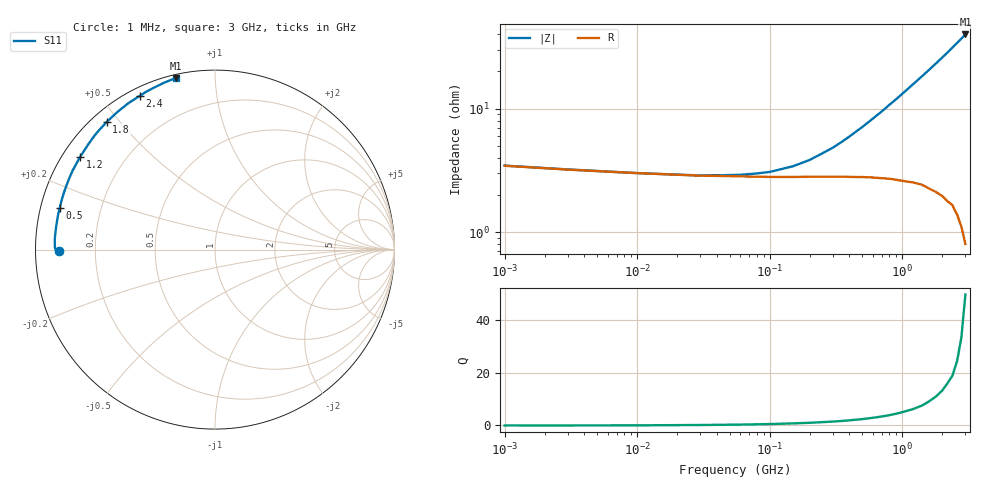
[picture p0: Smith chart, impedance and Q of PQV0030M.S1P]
! SIEMENS Small Signal Semiconductors
! BAR64-04
! Si PIN Diode in SOT23 (2 diodes in series, pin 3 open)
! IF = 30 mA
! S-Parameters:  July  1992
# GHz  S  MA  R  50
!  f  S11
! GHz  MAG  ANG
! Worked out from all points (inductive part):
!   33 points, 1 MHz to 3 GHz, reference 50 ohm
!   read as one part to ground: L = 2.05 nH near 700 MHz
!   highest Q = 49.8 at 3 GHz (marker M1), where L = 2.11 nH
!   S11 on the Smith chart (normalised r, x): 1 MHz: 0.07, -0.01; 500 MHz: 0.06, +0.13; 1.2 GHz: 0.05, +0.31; 1.8 GHz: 0.04, +0.46; 2.4 GHz: 0.03, +0.62; 3 GHz: 0.02, +0.80
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0.001  0.8712 -179.4
0.003  0.8796 -179.4
0.01  0.8868 -179.8
0.03  0.8918 179.4
0.08  0.8937 177.7
0.15  0.8944 175.5
0.2  0.8941 174.0
0.25  0.8941 172.4
0.3  0.8942 171.0
0.4  0.8952 168.0
0.45  0.8957 166.5
0.5  0.896 165.1
0.6  0.8976 162.2
0.7  0.8996 159.4
0.8  0.9015 156.5
0.9  0.9042 153.8
1  0.9071 151.0
1.2  0.9119 145.6
1.4  0.9177 140.4
1.5  0.9219 137.8
1.6  0.926 135.3
1.8  0.9328 130.3
2  0.9399 125.4
2.2  0.9477 120.7
2.4  0.9537 116.0
2.5  0.959 113.7
2.8  0.9719 107.1
3  0.9806 102.9
